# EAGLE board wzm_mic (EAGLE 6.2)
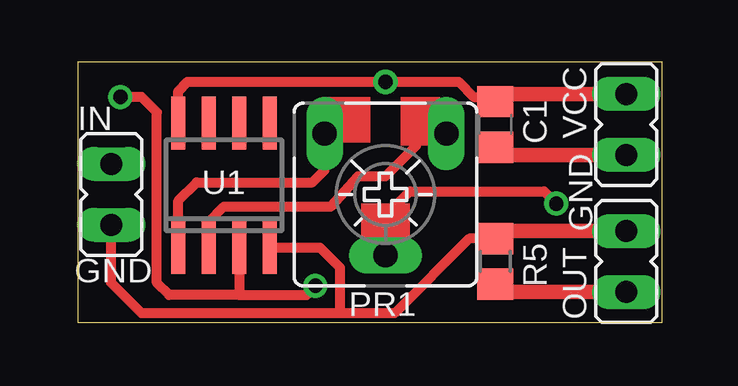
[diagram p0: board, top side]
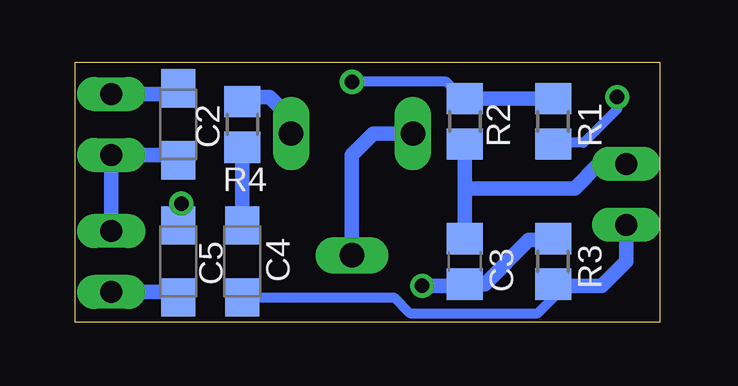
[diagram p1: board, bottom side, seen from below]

Size 24.36 x 10.85 mm. Coordinates in mm from the lower left corner, seen from the top.
Outline: 0,0 24.36,0 24.36,10.85 0,10.85 0,0
Copper layers (1*16): Top 0.035mm / dielectric 1.5mm / Bottom 0.035mm
Design rules: minimum track width 10mil, minimum drill 24mil, track to track 8mil, track to pad 8mil, pad to pad 8mil, via to via 8mil, smd to smd 8mil, copper to edge 40mil, drill to drill 8mil, minimum pad ring 10mil, minimum via ring 8mil, stop-mask expansion 4mil, vias tented up to drill 0mil, thermal gap 10mil

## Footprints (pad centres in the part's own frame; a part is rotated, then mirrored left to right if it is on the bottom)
C0805 = smd 1.3 x 1.5: 1 -0.95,0; 2 0.95,0
SMC_A = smd 1.6 x 1.4: + -1.5,0; - 1.5,0
JP1 = drill 0.914 long: 1 0,-1.27; 2 0,1.27
CA6V = drill 1.016 long: A -2.54,-2.54; E 2.54,-2.54; S 0,2.54
R0805 = smd 1.3 x 1.5: 1 -0.95,0; 2 0.95,0
SO08 = smd 0.6 x 2.2: 1 -1.905,-2.6; 2 -0.635,-2.6; 3 0.635,-2.6; 4 1.905,-2.6; 5 1.905,2.6; 6 0.635,2.6; 7 -0.635,2.6; 8 -1.905,2.6

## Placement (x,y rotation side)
C1  100nF  [C0805]  17.4,8.26 270 top
C2  10uF  [SMC_A]  20.07,8.26 270 bottom
C3  100nF  [C0805]  8.13,2.54 270 bottom
C4  10uF  [SMC_A]  17.4,2.54 270 bottom
C5  10uF  [SMC_A]  20.07,2.54 270 bottom
IN  [JP1]  1.4,5.33 0 top
OUT  [JP1]  22.86,2.54 0 top
PR1  [CA6V]  12.83,5.33 180 top
R1  100k  [R0805]  4.44,8.38 90 bottom
R2  4,7k  [R0805]  8.13,8.38 90 bottom
R3  100k  [R0805]  4.44,2.54 90 bottom
R4  1k  [R0805]  17.4,8.26 270 bottom
R5  100k  [R0805]  17.4,2.54 90 top
U1  TL072D  [SO08]  6.1,5.71 0 top
VCC  [JP1]  22.86,8.26 180 top

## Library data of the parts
C1-C5 R1-R5 = rcl
IN OUT VCC = jumper
PR1 = pot
U1 = linear

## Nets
GND: C1.2 C2.- C4.- IN.1 OUT.2 R3.1 R5.2 U1.4 VCC.2
N$1: C3.2 R1.1 R3.2 U1.3
N$2: C1.1 C2.+ R1.2 R2.2 U1.8 VCC.1
N$3: PR1.A R4.1 U1.2
N$4: C4.+ R4.2
N$5: C5.+ PR1.E PR1.S U1.1
N$6: C3.1 IN.2 R2.1
N$7: C5.- OUT.1 R5.1

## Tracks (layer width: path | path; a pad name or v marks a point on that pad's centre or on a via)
GND
  Top 0.406: 17.46,6.99 C1.2 | 17.72,3.81 R5.2 16.32,3.49 13.21,0.38 10.92,0.38 | U1.4 10.09,3.12 10.92,2.29 10.92,0.38 | 10.92,0.38 2.67,0.38 1.4,1.65 IN.1
  Top 0.61: VCC.2 17.46,6.99 | OUT.2 17.72,3.81
  Bottom 0.406: 19.79,6.99 C2.- 19.56,7.11 | 3.87,1.52 R3.1 3.94,1.52 5.08,0.38 10.41,0.38 11.05,1.02 17.38,1.02 C4.-
  Bottom 0.61: 19.79,6.99 VCC.2 OUT.2 | IN.1 1.4,2.54 2.41,1.52 3.87,1.52
N$1  (via drill 0.6)
  Top 0.406: U1.3 6.73,1.14 | 6.73,1.14 3.81,1.14 3.3,1.65 3.3,8.76 2.67,9.4 v1.78,9.4 | 6.73,1.14 9.53,1.14 v9.91,1.52
  Bottom 0.406: 4,3.43 R3.2 | v1.78,9.4 1.78,8.89 3.17,7.49 4.38,7.49 R1.1 | 8.19,1.52 C3.2
  Bottom 0.61: C3.2 7.3,1.59 5.46,3.43 4,3.43 | v9.91,1.52 8.19,1.52
N$2  (via drill 0.6)
  Top 0.406: 17.34,9.53 C1.1 17.59,9.4 16.51,9.4 15.88,10.03 v12.83,10.03 4.57,10.03 4.19,9.65 U1.8
  Top 0.61: VCC.1 17.34,9.53
  Bottom 0.406: 20.04,9.53 C2.+ | R2.2 8.19,9.33 8.89,10.03 v12.83,10.03
  Bottom 0.61: VCC.1 20.04,9.53 | R1.2 R2.2
N$3
  Top 0.406: U1.2 5.46,4.19 6.1,4.83 10.54,4.83 11.68,6.1 12.83,6.1 14.1,7.37 14.1,7.87 | 14.1,7.87 13.84,7.87 | 14.1,7.87 PR1.A
  Bottom 0.406: 17.33,9.4 R4.1
  Bottom 0.61: PR1.A 15.37,8.51 16.26,9.4 17.33,9.4
N$4
  Bottom 0.61: R4.2 C4.+
N$5  (via drill 0.6)
  Top 0.406: U1.1 4.19,5.08 4.95,5.84 9.78,5.84 10.29,6.35 PR1.E | PR1.S 12.83,4.45 13.84,5.46 19.43,5.46 v19.94,4.95
  Bottom 0.406: v19.94,4.95 19.91,4.06 C5.+
  Bottom 0.61: PR1.E 11.94,7.87 12.83,6.99 PR1.S
N$6
  Bottom 0.61: IN.2 2.54,6.6 3.56,5.59 8.13,5.59 | 8.13,5.59 C3.1 | R2.1 8.13,5.59
N$7
  Top 0.406: 17.59,1.27 R5.1
  Top 0.61: OUT.1 17.59,1.27
  Bottom 0.406: 19.91,1.27 C5.-
  Bottom 0.61: OUT.1 19.91,1.27
(copper drawn outside any net)
  shapes: Top area x3

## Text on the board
tNames: GND | GND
